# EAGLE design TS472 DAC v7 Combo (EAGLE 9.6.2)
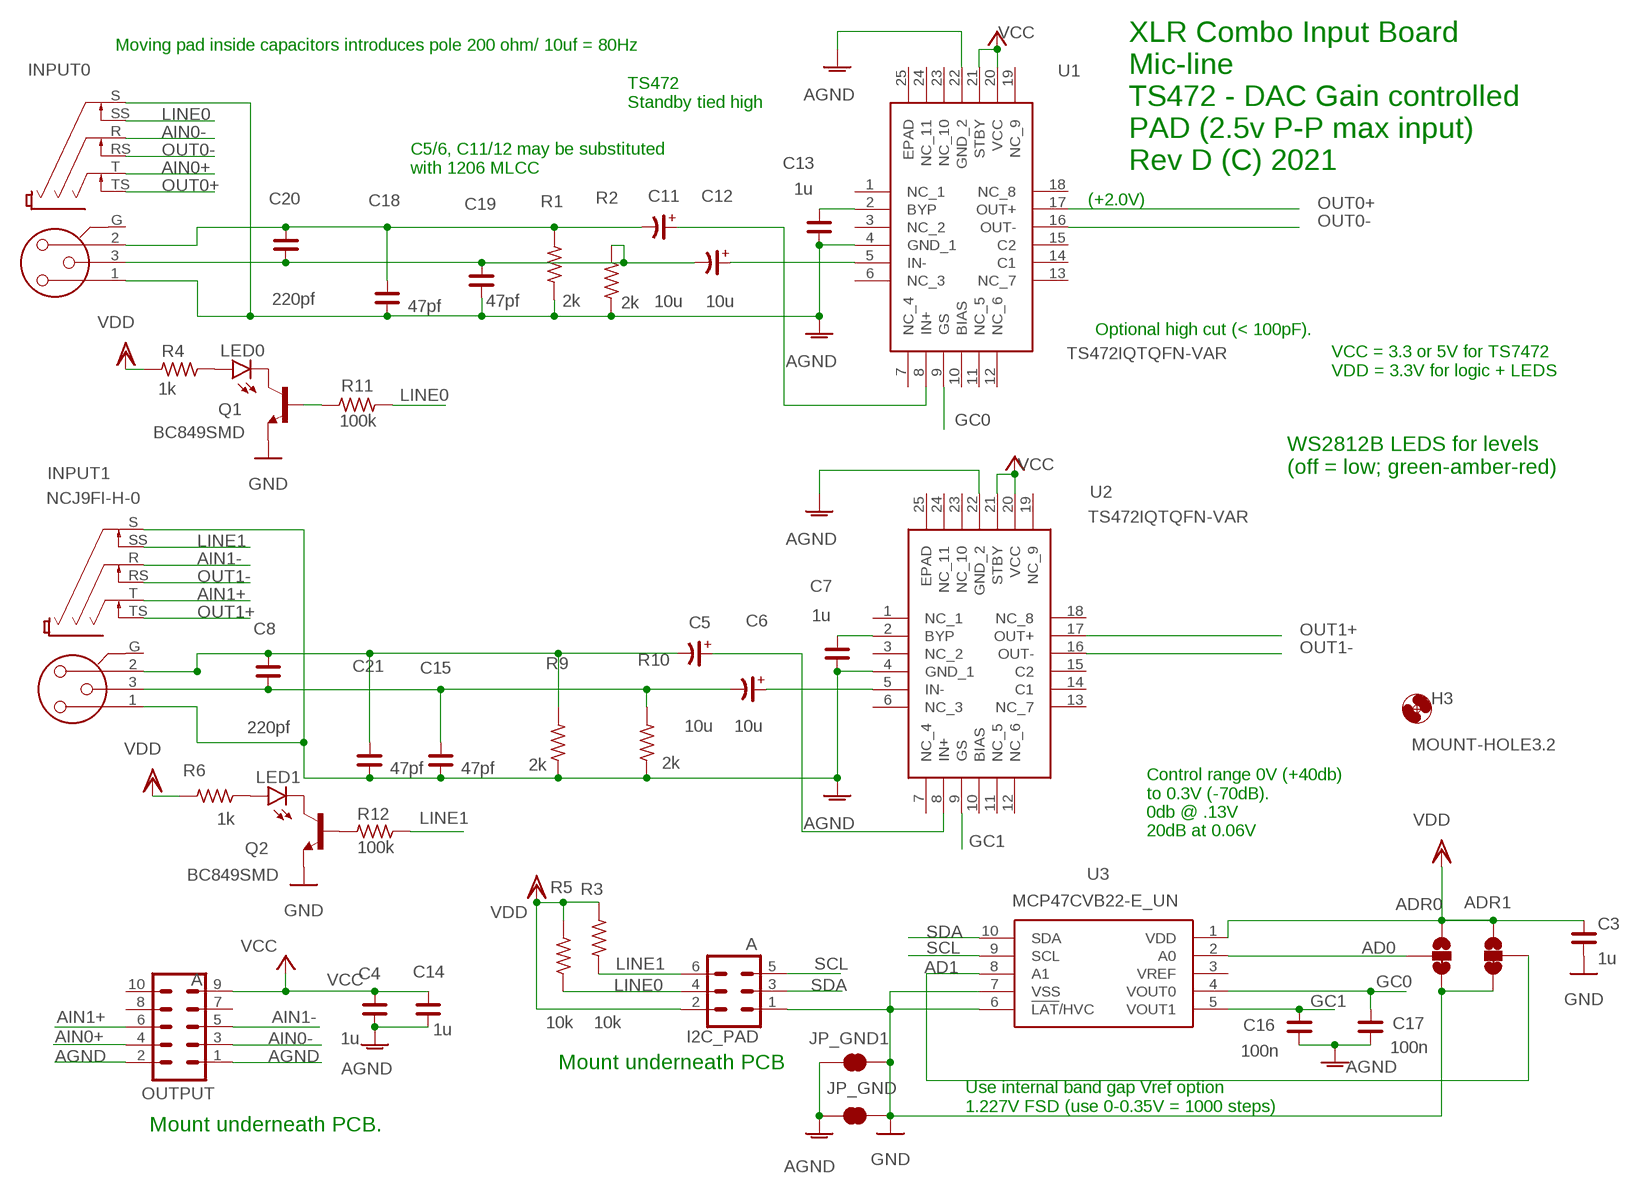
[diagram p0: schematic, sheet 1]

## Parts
ADR0  JUMPER-SMT_3_1-NC_TRACE_SILK  [SMT-JUMPER_3_1-NC_TRACE_SILK]
ADR1  JUMPER-SMT_3_1-NC_TRACE_SILK  [SMT-JUMPER_3_1-NC_TRACE_SILK]
C3  1u  C_0805  [C0805]
C4  1u  C_0805  [C0805]
C5  10u  CP_SV-B  [CSV-B]
C6  10u  CP_SV-B  [CSV-B]
C7  1u  C_0805  [C0805]
C8  220pf  C_0805  [C0805]
C11  10u  CP_SV-B  [CSV-B]
C12  10u  CP_SV-B  [CSV-B]
C13  1u  C_0805  [C0805]
C14  1u  C_0805  [C0805]
C15  47pf  C_0805  [C0805]
C16  100n  C_0805  [C0805]
C17  100n  C_0805  [C0805]
C18  47pf  C_0805  [C0805]
C19  47pf  C_0805  [C0805]
C20  220pf  C_0805  [C0805]
C21  47pf  C_0805  [C0805]
H3  MOUNT-HOLE3.2  [3,2]
I2C_PAD  A  CONN_03X2SHROUD  [2X3-SHROUDED]
INPUT0  NCJ9FI-H-0  [NCJ9FI-H]
INPUT1  NCJ9FI-H-0  [NCJ9FI-H]
JP_GND  JUMPER-SMT_2_NC_TRACE_NO-SILK  [SMT-JUMPER_2_NC_TRACE_NO-SILK]
JP_GND1  JUMPER-SMT_2_NC_TRACE_NO-SILK  [SMT-JUMPER_2_NC_TRACE_NO-SILK]
LED0  LG_T679-E1F1-1  [PLCC2]
LED1  LG_T679-E1F1-1  [PLCC2]
OUTPUT  A  CONN_05X2SHD_LOCK  [2X5-SHROUDED_LOCK]
Q1  BC849SMD  [SOT23-BEC]
Q2  BC849SMD  [SOT23-BEC]
R1  2k  R_0805  [R0805]
R2  2k  R_0805  [R0805]
R3  10k  R_0805  [R0805]
R4  1k  R_0805  [R0805]
R5  10k  R_0805  [R0805]
R6  1k  R_0805  [R0805]
R9  2k  R_0805  [R0805]
R10  2k  R_0805  [R0805]
R11  100k  R_0805  [R0805]
R12  100k  R_0805  [R0805]
U1  TS472IQTQFN-VAR  [QFN50P400X400X100-25N-VAR]
U2  TS472IQTQFN-VAR  [QFN50P400X400X100-25N-VAR]
U3  MCP47CVB22-E_UN  [SOP50P490X110-10N]

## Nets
AD0: ADR0.2 U3.2(A0)
AD1: ADR1.2 U3.8(A1)
AGND: C4.1 C7.1 C13.1 C14.1 C15.1 C16.1 C17.1 C18.1 C19.1 C21.1 INPUT0.1 INPUT0.S INPUT1.1 INPUT1.S JP_GND1.1 JP_GND.1 OUTPUT.1 OUTPUT.2 R1.1 R2.1 R9.1 R10.1 U1.4(GND_1) U1.22(GND_2) U2.4(GND_1) U2.22(GND_2)
AIN0+: INPUT0.T OUTPUT.4
AIN0-: INPUT0.R OUTPUT.3
AIN1+: INPUT1.T OUTPUT.6
AIN1-: INPUT1.R OUTPUT.5
GC0: C17.2 U1.9(GS) U3.4(VOUT0)
GC1: C16.2 U2.9(GS) U3.5(VOUT1)
GND: ADR0.3 ADR1.3 C3.1 I2C_PAD.1 JP_GND1.2 JP_GND.2 Q1.E Q2.E U3.6(!LAT!/HVC) U3.7(VSS)
LINE0: I2C_PAD.4 INPUT0.SS R5.2 R11.2
LINE1: I2C_PAD.6 INPUT1.SS R3.2 R12.2
N$1: C6.- C8.1 C15.2 INPUT1.3 R10.2
N$3: C11.+ U1.8(IN+)
N$4: C5.+ U2.8(IN+)
N$5: C13.2 U1.2(BYP)
N$8: C12.+ U1.5(IN-)
N$10: C11.- C18.2 C20.2 INPUT0.2 R1.2
N$11: C12.- C19.2 C20.1 INPUT0.3 R2.2
N$13: LED0.A R4.1
N$17: LED1.A R6.1
N$20: Q1.B R11.1
N$21: C7.2 U2.2(BYP)
N$24: C5.- C8.2 C21.2 INPUT1.2 R9.2
N$25: Q2.B R12.1
N$26: LED1.C Q2.C
N$27: C6.+ U2.5(IN-)
N$28: LED0.C Q1.C
OUT0+: INPUT0.TS U1.17(OUT+)
OUT0-: INPUT0.RS U1.16(OUT-)
OUT1+: INPUT1.TS U2.17(OUT+)
OUT1-: INPUT1.RS U2.16(OUT-)
SCL: I2C_PAD.5 U3.9(SCL)
SDA: I2C_PAD.3 U3.10(SDA)
VCC: C4.2 C14.2 OUTPUT.9 U1.20(VCC) U1.21(STBY) U2.20(VCC) U2.21(STBY)
VDD: ADR0.1 ADR1.1 C3.2 I2C_PAD.2 R3.1 R4.2 R5.1 R6.2 U3.1(VDD)
Unconnected: INPUT0.G INPUT1.G OUTPUT.7 OUTPUT.8 OUTPUT.10 U1.1(NC_1) U1.3(NC_2) U1.6(NC_3) U1.7(NC_4) U1.10(BIAS) U1.11(NC_5) U1.12(NC_6) U1.13(NC_7) U1.14(C1) U1.15(C2) U1.18(NC_8) U1.19(NC_9) U1.23(NC_10) U1.24(NC_11) U1.25(EPAD) U2.1(NC_1) U2.3(NC_2) U2.6(NC_3) U2.7(NC_4) U2.10(BIAS) U2.11(NC_5) U2.12(NC_6) U2.13(NC_7) U2.14(C1) U2.15(C2) U2.18(NC_8) U2.19(NC_9) U2.23(NC_10) U2.24(NC_11) U2.25(EPAD) U3.3(VREF)

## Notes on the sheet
- Moving pad inside capacitors introduces pole 200 ohm/ 10uf = 80Hz
- TS472
  Standby tied high
- XLR Combo Input Board
  Mic-line 
  TS472 - DAC Gain controlled
  PAD (2.5v P-P max input)
  Rev D (C) 2021
- C5/6, C11/12 may be substituted 
  with 1206 MLCC
- (+2.0V)
- Optional high cut (< 100pF).
- VCC = 3.3 or 5V for TS7472
  VDD = 3.3V for logic + LEDS
- WS2812B LEDS for levels
  (off = low; green-amber-red)
- Control range 0V (+40db) 
  to 0.3V (-70dB). 
  0db @ .13V
  20dB at 0.06V
- Mount underneath PCB
- Use internal band gap Vref option
  1.227V FSD (use 0-0.35V = 1000 steps)
- Mount underneath PCB.

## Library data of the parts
ADR0 ADR1 = MY-SparkFun-Jumpers:JUMPER-SMT_3_1-NC_TRACE: Normally closed trace jumper (1 of 2 connections) This jumper has a trace between two pads so it's normally closed (NC). The other connection is normally open (NO). Use a razor knife to open the connection. For best results follow the IPC guidelines for cutting traces: Cutout at least 0.063 mm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
C3 C4 C7 C8 C13-C21 = rc-master-smd:C_: NON-POLARIZED CAP
C5 C6 C11 C12 = rc-master-smd:CP_: POLARIZED CAP
H3 = holes:MOUNT-HOLE: MOUNTING HOLE with drill center marker
I2C_PAD = SparkFun-Connectors:CONN_03X2: Multi connection point. Often used as Generic Header-pin footprint for 0.1 inch spaced/style header connections You can populate with any combo of single row headers, but if you'd like an exact match, check these: Header - 2x3 (Male, 0.1") (PRT-12807) Header - 2x3 (Female, 0.1") (PRT-13010) 2x3 Pin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; PROD_ID: CONN-10681; SF_ID: PRT_10877
INPUT0 INPUT1 = con-neutrik_xlr_2:NCJ9FI: NCJ9FI Combination - 3 pin Female XLR - 3 pin 1/4" switched socket Combo I series Without or without retention latch Source: www.neutrik.com/
JP_GND JP_GND1 = MY-SparkFun-Jumpers:JUMPER-SMT_2_NC_TRACE: Normally closed trace jumper
LED0 LED1 = led:*_T679-?-1: LC TOPLED® Low Current LED; COLOR: green
OUTPUT = SparkFun-Connectors:CONN_05X2: Multi connection point. Often used as Generic Header-pin footprint for 0.1 inch spaced/style header connections For AVR SPI programming port, see special device with nice symbol: "AVR_SPI_PROG_5x2.dev" You can populate with any combo of single row headers, but if you'd like an exact match, check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; PROD_ID: CONN-08671; SF_ID: PRT-08506
Q1 Q2 = transistor-npn:BC849*: NPN Transistor
R1-R6 R9-R12 = rc-master-smd:R_: RESISTOR
U1 U2 = SamacSys_Parts:TS472IQT: STMICROELECTRONICS - TS472IQT - AMPLIFIER, CLASS AB, QFN-24 Source: Datasheet
U3 = SamacSys_Parts:MCP47CVB22-E_UN: Digital to Analog Converters - DAC I2C, Dual Channel, 12-Bit, Volatile Source: Datasheet; DESCRIPTION: Digital to Analog Converters - DAC I2C, Dual Channel, 12-Bit, Volatile; HEIGHT: 1.1mm; MANUFACTURER_NAME: Microchip; MANUFACTURER_PART_NUMBER: MCP47CVB22-E/UN; MOUSER_PART_NUMBER: 579-MCP47CVB22-E/UN; MOUSER_PRICE-STOCK: https://www.mouser.co.uk/ProductDetail/Microchip-Technology/MCP47CVB22-E-UN/?qs=byeeYqUIh0PPQDcqck%252Boaw%3D%3D

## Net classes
0 default: width 0.152 mm
3 power: width 0.305 mm

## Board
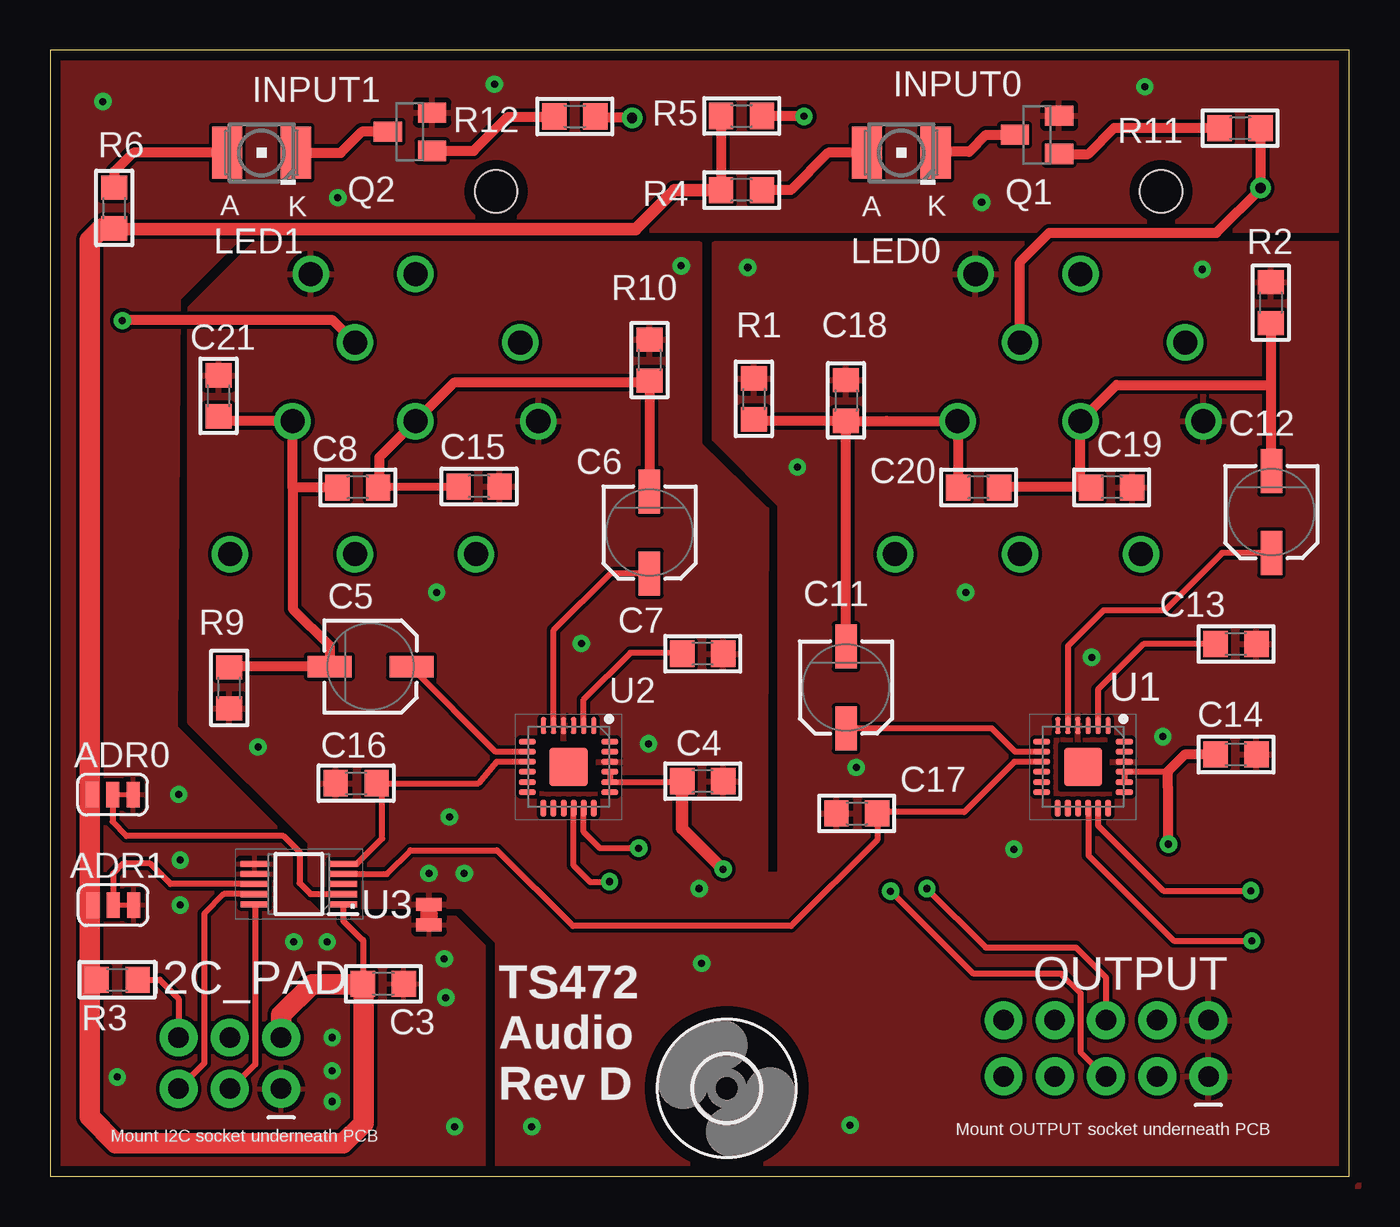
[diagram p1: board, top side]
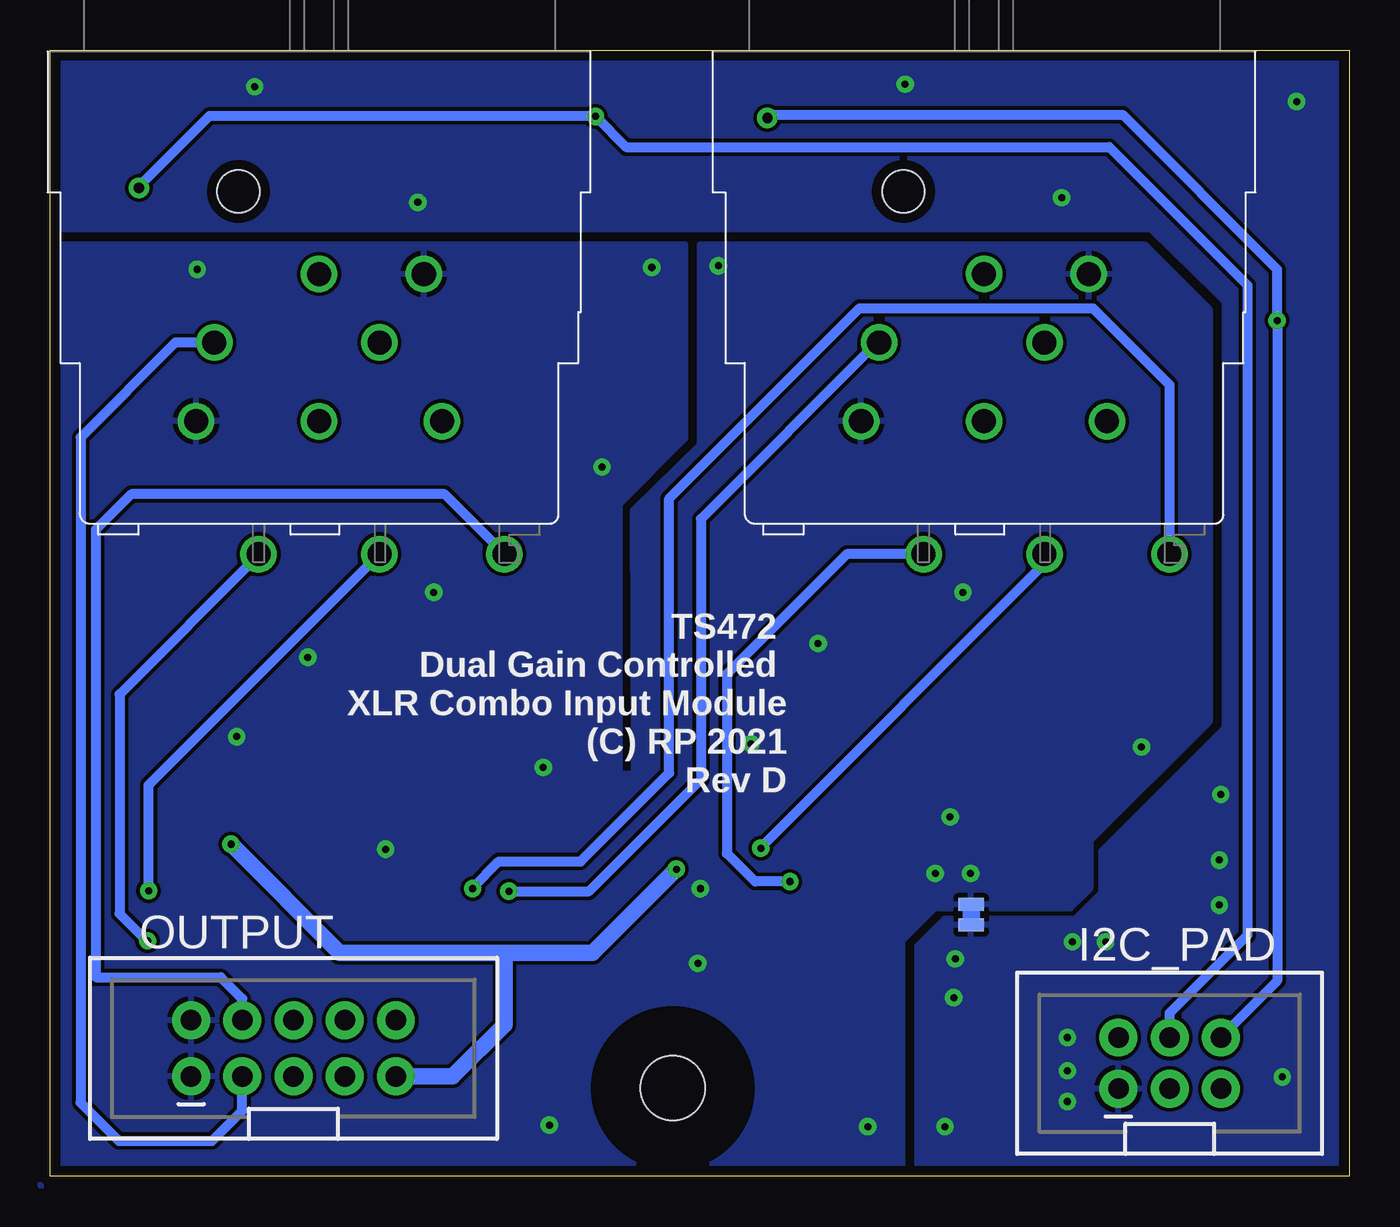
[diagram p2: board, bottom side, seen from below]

Size 64.45 x 55.88 mm. Coordinates in mm from the lower left corner, seen from the top.
Outline: 0,55.88 0,0 64.46,0 64.46,55.88 0,55.88
Copper layers (1*16): Top 0.035mm / dielectric 1.5mm / Bottom 0.035mm
Design rules "SparkFun - PCBWAY": minimum track width 8mil, minimum drill 13.5mil, track to track 7mil, track to pad 7mil, pad to pad 7mil, via to via 7mil, smd to smd 8mil, copper to edge 20mil, drill to drill 8mil, minimum pad ring 12mil, minimum via ring 10mil, stop-mask expansion 4mil, vias tented up to drill 25mil, thermal gap 10mil

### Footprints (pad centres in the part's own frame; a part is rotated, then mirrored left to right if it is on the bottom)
SMT-JUMPER_3_1-NC_TRACE_SILK = smd 0.635 x 1.27: 1 -1.016,0; 2 0,0; 3 1.016,0
C0805 = smd 1.2 x 1.3: 1 -1.016,0; 2 1.016,0
CSV-B = smd 2.184 x 1.067: + -2.032,0; - 2.032,0
3,2 = hole 3.2: 0,0
2X3-SHROUDED = drill 1.016 pad 1.88: 1 -1.27,2.54; 2 1.27,2.54; 3 -1.27,0; 4 1.27,0; 5 -1.27,-2.54; 6 1.27,-2.54
NCJ9FI-H = drill 1.2: 1 -6.1,-18.4; 2 6.1,-18.4; 3 0,-18.4; G 0,-11.1; R -5.2,-14.5; RS -3,-25; S 5.2,-11.1; SS 3,-14.5; T 9.2,-25; TS 3,-25 | hole 2.1: -4,-7
SMT-JUMPER_2_NC_TRACE_NO-SILK = smd 0.635 x 1.27: 1 -0.508,0; 2 0.508,0
PLCC2 = smd 2.6 x 1.5: A 0,1.7; C 0,-1.7
2X5-SHROUDED_LOCK = drill 1.016 pad 1.88: 1 -1.397,5.08; 2 1.397,5.08; 3 -1.397,2.54; 4 1.397,2.54; 5 -1.397,0; 6 1.397,0; 7 -1.397,-2.54; 8 1.397,-2.54; 9 -1.397,-5.08; 10 1.397,-5.08
SOT23-BEC = smd 1 x 1.4: B -0.95,-1.1; C 0,1.1; E 0.95,-1.1
R0805 = smd 1.2 x 1.3: 1 -1.016,0; 2 1.016,0
QFN50P400X400X100-25N-VAR = smd 0.838 x 0.254: 1 -2.052,1.25; 2 -2.052,0.75; 3 -2.052,0.25; 4 -2.052,-0.25; 5 -2.052,-0.75; 6 -2.052,-1.25 | smd 0.3 x 0.85: 7 -1.25,-2.052; 8 -0.75,-2.052; 9 -0.25,-2.052; 10 0.25,-2.052; 11 0.75,-2.052; 12 1.25,-2.052; 19 1.25,2.052; 20 0.75,2.052; 21 0.25,2.052; 22 -0.25,2.052; 23 -0.75,2.052; 24 -1.25,2.052 | smd 0.85 x 0.3: 13 2.052,-1.25; 14 2.052,-0.75; 15 2.052,-0.25; 16 2.052,0.25; 17 2.052,0.75; 18 2.052,1.25 | smd 1.905 x 1.905: 25 0,0
SOP50P490X110-10N = smd 1.4 x 0.3: 1 -2.2,1; 2 -2.2,0.5; 3 -2.2,0; 4 -2.2,-0.5; 5 -2.2,-1; 6 2.2,-1; 7 2.2,-0.5; 8 2.2,0; 9 2.2,0.5; 10 2.2,1

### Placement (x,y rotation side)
ADR0  3.09,18.95 0 top
ADR1  3.11,13.46 0 top
C3  16.53,9.55 180 top
C4  32.37,19.61 180 top
C5  15.89,25.3 180 top
C6  29.73,31.95 90 top
C7  32.37,25.93 180 top
C8  15.26,34.19 180 top
C11  39.49,24.26 90 top
C12  60.59,32.97 90 top
C13  58.84,26.42 180 top
C14  58.84,20.93 180 top
C15  21.27,34.24 180 top
C16  15.18,19.51 0 top
C17  40.02,18.01 0 top
C18  39.49,38.51 270 top
C19  52.67,34.19 180 top
C20  46.07,34.19 180 top
C21  8.35,38.73 270 top
H3  33.57,4.37 270 top
I2C_PAD  8.91,5.61 90 bottom
INPUT0  51.12,55.88 0 bottom
INPUT1  18.12,55.88 0 bottom
JP_GND  18.79,12.98 270 top
JP_GND1  18.76,12.98 270 bottom
LED0  42.23,50.8 90 top
LED1  10.48,50.8 90 top
OUTPUT  52.39,6.35 90 bottom
Q1  48.96,51.69 90 top
Q2  17.85,51.84 90 top
R1  34.91,38.58 270 top
R2  60.57,43.36 270 top
R3  3.32,9.75 0 top
R4  34.31,48.95 180 top
R5  34.31,52.63 0 top
R6  3.16,48.06 270 top
R9  8.88,24.23 90 top
R10  29.73,40.51 270 top
R11  59.04,52.02 0 top
R12  26.02,52.6 0 top
U1  51.25,20.32 270 top
U2  25.72,20.32 270 top
U3  12.33,14.5 180 top

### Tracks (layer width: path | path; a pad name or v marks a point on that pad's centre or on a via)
AD0
  Top 0.305: ADR0.2 3.09,17.59 3.77,16.89 11.57,16.89 12.36,16.1 12.36,14.55 12.91,14 U3.2
AD1
  Top 0.305: U3.8 5.97,14.5 4.95,15.52 3.62,15.52 3.11,15.01 ADR1.2
AGND  (via drill 0.35)
  other vias: 29.68,21.46 57.17,45.01 34.61,45.11 19.17,28.98 20.54,15.04 39.69,2.54 37.07,35.2 19.8,17.83 45.43,28.98 47.82,16.23 55.21,21.82 26.36,26.44 51.68,25.76 10.3,21.31 23.89,2.46 18.79,15.04 32.2,14.27 32.32,10.57 39.99,20.29 31.31,45.19
  pour Top: 64.93,46.25 32.96,46.25 32.96,36.6 36.21,33.35 36.21,14.96 35.5,14.96 35.5,20.85 35.55,33.07 32.22,36.32 32.22,46.25 10.15,46.25 6.92,43.03 6.92,22.56 12.89,16.59 12.89,14.45 13.93,13.41 20.44,13.41 22.19,11.66 22.19,-0.45 64.93,-0.5
  pour Bottom: 64.93,46.25 32.96,46.25 32.96,36.6 36.21,33.35 36.21,19.99 35.5,19.99 35.5,20.85 35.55,33.07 32.22,36.32 32.22,46.25 10.15,46.25 6.92,43.03 6.92,22.56 12.84,16.64 12.84,14.27 13.83,13.28 20.56,13.28 22.19,11.66 22.19,-0.45 64.93,-0.5
  cutout Top: 24.5,21.54 26.99,21.54 26.99,19.15 24.5,19.15
  cutout Top: 50.1,21.49 52.49,21.49 52.49,19.15 50.1,19.15
AIN0+
  Bottom 0.508: INPUT0.T 44.9,33.86 60.44,33.86 62.19,32.11 62.19,9.88 56,9.88 54.93,8.81 OUTPUT.4
AIN0-
  Bottom 0.508: INPUT0.R 58.25,41.38 62.96,36.67 62.96,3.66 61.05,1.75 56.43,1.75 54.93,3.25 OUTPUT.3
AIN1+  (via drill 0.35)
  Top 0.305: v43.5,14.27 46.42,11.35 50.9,11.35 52.39,9.87 OUTPUT.6
  Bottom 0.508: v43.5,14.27 43.5,14.33 42.2,15.62 38.14,15.62 33.75,20.02 33.75,33.63 24.3,43.08 12.71,43.08 8.92,39.28 INPUT1.T
AIN1-  (via drill 0.35)
  Top 0.305: 41.72,14.15 45.81,10.06 50.16,10.06 51.12,9.09 51.12,6.18 52.35,4.95 OUTPUT.5
  Top 0.508: v41.7,14.15 41.72,14.15
  Bottom 0.508: v41.7,14.15 37.73,14.15 32.17,19.71 32.17,32.63 23.42,41.38 INPUT1.R
GC0
  Top 0.305: U1.9 47.84,20.57 45.35,18.08 41.11,18.08 C17.2 41.04,16.69 36.77,12.42 25.93,12.42 22.17,16.18 17.87,16.18 16.7,15 U3.4
GC1
  Top 0.305: U2.9 22.15,20.57 21.25,19.51 C16.2 16.46,19.51 16.46,16.76 15.2,15.5 U3.5
GND  (via drill 0.35)
  other vias: 22.04,54.2 54.32,54.08 2.61,53.34 6.37,18.95 13.99,3.71 46.22,48.34 13.99,5.23 13.99,6.88 3.32,4.93 14.26,48.56 6.44,13.46 19.55,10.79 6.44,15.7 19.62,8.86 20.06,2.46 12.08,11.63 13.73,11.63
  pour Top: -0.39,56.01 6.21,56.01 6.21,55.93 9.77,52.37 9.77,46.94 6.36,43.53 6.21,22.3 12.36,16.15 12.36,14.07 13.58,12.85 20.08,12.85 21.5,11.43 21.5,-0.48 -0.39,-0.48
  pour Top (rank 2): -0.57,56.77 -0.57,41.78 3.83,41.78 9.03,46.99 65.24,46.99 65.24,56.77
  pour Bottom: -0.95,59.05 6.19,59.05 6.19,22.25 12.31,16.13 12.31,14.07 13.6,12.78 20.08,12.78 21.45,11.4 21.45,-0.89 -0.95,-0.89
  pour Bottom (rank 2): -1.46,57.53 -1.46,41.78 4.52,41.78 9.84,46.99 65.65,46.99 65.65,57.53
LINE0  (via drill 0.35, 0.51)
  Top 0.508: R11.2 v60.06,49.05 60.06,49.01 57.88,46.82 49.57,46.82 48.12,45.37 INPUT0.SS | R5.2 37.4,52.63 v37.4,52.6
  Bottom 0.508: v60.06,49.05 60.1,49.09 56.56,52.63 37.4,52.63 v37.4,52.6 35.88,51.08 11.9,51.08 5.04,44.22 5.04,11.96 8.91,8.1 I2C_PAD.4
LINE1  (via drill 0.35, 0.51)
  Top 0.305: R3.2 5.43,9.75 6.37,8.81 I2C_PAD.6
  Top 0.406: v3.57,42.47 3.41,42.48
  Top 0.508: v28.87,52.53 26.98,52.53 R12.2 | 3.41,42.48 14.02,42.48 INPUT1.SS
  Bottom 0.508: v28.87,52.53 28.72,52.68 11.24,52.68 3.57,45.01 v3.57,42.47 3.57,9.7 6.37,6.91 I2C_PAD.6
N$1
  Top 0.406: C8.1 16.32,34.24 C15.2
  Top 0.508: 16.32,34.24 16.32,35.68 INPUT1.3 20.03,39.39 29.63,39.39 R10.2 C6.-
N$3
  Top 0.305: U1.8 47.88,21.07 46.72,22.23 39.5,22.23 C11.+
N$4
  Top 0.305: U2.8 22.1,21.07 17.87,25.3 C5.+
N$5
  Top 0.305: C13.2 54.24,26.42 52,24.17 U1.2
N$8
  Top 0.305: C12.+ 58.16,30.94 55.31,28.09 52.26,28.09 50.5,26.33 U1.5
N$10
  Top 0.203: INPUT0.2 45.05,37.45
  Top 0.508: INPUT0.2 41.5,37.48 41.49,37.49 C18.2 | 45.05,37.45 C20.2 | C18.2 34.99,37.49 R1.2 | C11.- C18.2
N$11
  Top 0.508: C20.1 47.11,34.21 51.63,34.21 C19.2 51.12,34.19 51.09,34.21 51.09,37.45 INPUT0.3 52.91,39.27 60.57,39.27 | C12.- 60.57,35.03 60.57,39.27 | R2.2 60.57,39.27
N$13
  Top 0.508: LED0.A 38.6,50.8 36.75,48.95 R4.1
N$17
  Top 0.508: LED1.A 4.1,50.8 3.17,49.86 R6.1
N$20
  Top 0.508: Q1.B 51.51,50.74 52.79,52.02 R11.1
N$21
  Top 0.305: U2.2 26.47,23.66 28.79,25.98 31.31,25.98 C7.2
N$24
  Top 0.508: C21.2 8.59,37.48 INPUT1.2 12.02,34.19 C8.2 12.03,34.19 12.03,28.17 13.86,26.34 C5.- 8.93,25.3 R9.2
N$25
  Top 0.508: R12.1 24.99,52.56 22.67,52.56 21,50.89 Q2.B
N$26
  Top 0.508: Q2.C 15.46,51.84 14.42,50.8 LED1.C
N$27
  Top 0.305: C6.+ 27.8,29.92 24.98,27.1 24.98,22.39 U2.5
N$28
  Top 0.508: Q1.C 46.44,51.69 45.6,50.85 43.98,50.85 LED0.C
OUT0+  (via drill 0.35)
  Top 0.305: U1.17 52,17.41 55.08,14.33 55.21,14.2 55.24,14.17 v59.58,14.17
  Bottom 0.508: INPUT0.TS 59.58,19.42 v59.58,14.17
OUT0-  (via drill 0.35)
  Top 0.305: U1.16 51.51,18.25 51.51,15.92 55.75,11.68 v59.63,11.68
  Bottom 0.305: v59.63,11.68 59.68,11.68
  Bottom 0.508: 59.68,11.68 61.03,13.03 61.03,23.92 54.12,30.83 INPUT0.RS
OUT1+  (via drill 0.35)
  Top 0.305: 27.27,16.28 | v29.2,16.28 27.27,16.28 | 27.27,16.28 26.47,17.08 U2.17
  Bottom 0.406: v29.2,16.28 29.2,16.33 | 15.12,30.41 INPUT1.TS
  Bottom 0.508: 29.2,16.33 15.12,30.41
OUT1-  (via drill 0.35)
  Top 0.305: U2.16 25.97,15.42 26.8,14.59 27.72,14.59 v27.75,14.62
  Bottom 0.508: v27.75,14.62 29.48,14.62 30.88,16.02 30.88,24.93 24.93,30.88 INPUT1.RS
SCL
  Top 0.305: U3.9 8.61,14 7.64,13.03 7.64,5.61 I2C_PAD.5
SDA
  Top 0.305: U3.10 10.18,13.45 10.18,5.56 8.91,4.29 I2C_PAD.3
VCC  (via drill 0.35)
  Top 0.305: U1.20 U1.21 55.44,20.07 | U2.21 U2.20 31.38,19.57 C4.2
  Top 0.508: C14.2 56.3,20.93 55.44,20.07 55.46,20.04 55.46,19.28 55.46,18.95 55.46,16.51 v55.49,16.48
  Top 0.61: v33.39,15.24 31.36,17.27 C4.2
  Bottom 0.813: OUTPUT.9 44.49,4.95 41.93,7.52 41.93,11.1 | 41.93,11.1 50.1,11.1 v55.49,16.48 | 41.93,11.1 37.56,11.1 33.42,15.24 v33.39,15.24
VDD
  Top 0.305: U3.1 14.53,12.68 15.5,11.71 15.51,11.74 C3.2 | R3.1 2.25,9.75 1.95,10.06
  Top 0.406: ADR1.1 1.95,13.46
  Top 0.508: ADR0.1 1.95,17.58 1.95,16.41 | R5.1 33.29,49.2 33.04,48.95
  Top 0.61: R4.2 33.04,48.95 30.98,48.95 29.05,47.02 3.19,47.02 R6.2
  Top 1.016: R6.2 2.53,47.04 1.95,46.46 1.95,16.41 1.95,13.46 1.95,10.06 1.95,2.95 3.25,1.64 14.53,1.64 15.53,2.64 15.53,9.55 C3.2 15.49,9.53 12.98,9.53 11.45,8 I2C_PAD.2

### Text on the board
bPlace: TS472 / Dual Gain Controlled / XLR Combo Input Module / (C) RP 2021 / Rev D
tNames: A | K | A | K | . | I2C_PAD | OUTPUT | TS472 / Audio / Rev D | Mount OUTPUT socket underneath PCB | Mount I2C socket underneath PCB

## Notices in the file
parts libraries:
SparkFun-Connectors: Licensing: Creative Commons ShareAlike 4.0 International - https://creativecommons.org/licenses/by-sa/4.0
rc-master-smd: Copyright (C) 2007, Bob Starr
